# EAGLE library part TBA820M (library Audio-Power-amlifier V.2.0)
The TBA820M is a monolithic integrated audio amplifier in a 8 lead dual in-line plastic package. It is intended for use as low frequency class B power amplifier with wide range of supply voltage: 3 to 16V, in portable radios, cassette recorders and players etc. Main features are: minimum working supply voltage of 3V, low quiescent current, low number of external components, good ripple rejection, no cross-over distortion, low power dissipation. Output power: Po = 2Wat 12V/8W, 1.6W at 9V/4W and 1.2W at 9V/8W.
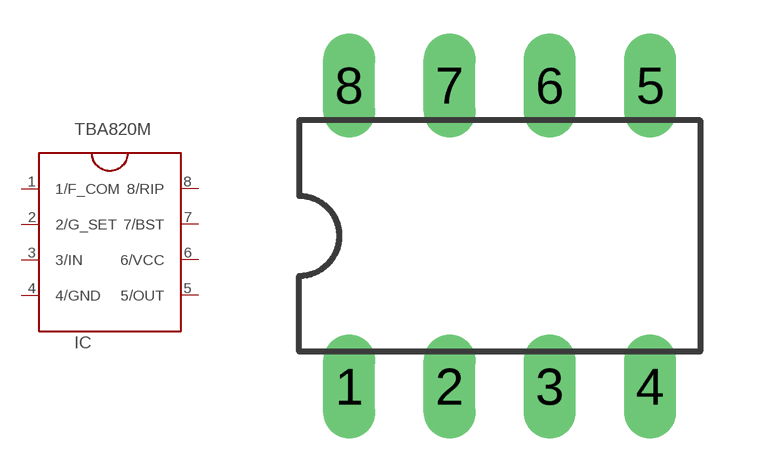
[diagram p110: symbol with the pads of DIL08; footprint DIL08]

Designator prefix IC

## TBA820M  [DIL08]
1  1/F_COM
2  2/G_SET
3  3/IN  in
4  4/GND  pwr
5  5/OUT  out
6  6/VCC  pwr
7  7/BST
8  8/RIP

## Footprint DIL08 (pad centres in mm)
Dual In Line Package
drill 0.813 pad 1.27 long: 1 -3.81,-3.81; 2 -1.27,-3.81; 3 1.27,-3.81; 4 3.81,-3.81; 5 3.81,3.81; 6 1.27,3.81; 7 -1.27,3.81; 8 -3.81,3.81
